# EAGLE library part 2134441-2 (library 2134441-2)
Body Features: Offset .88 MM | Shell Plating Material Tin over Nickel | Shell Plating Finish Matte | Connector Profile Micro | Configuration Features: Number of Positions 5 | Number of Ports 1 | Contact Features: Contact Mating Area Plating Material Thickness .76 MICM | Contact Current Rating (Max) 1.8 AMP | Contact Mating Area Plating Material Gold | Contact Mating Area Plating Material Thickness 29.52 MICIN | Dimensions: PCB Thickness (Recommended) .8 1. MM | PCB Thickness (Recommended) .031 .039 Source: Datasheet
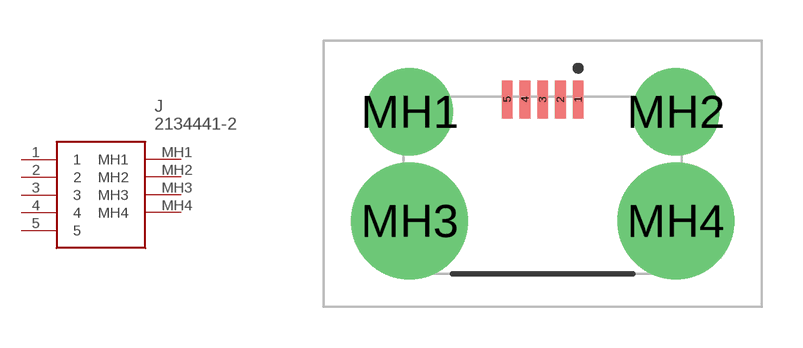
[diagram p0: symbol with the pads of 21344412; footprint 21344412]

Designator prefix J

## 2134441-2 (Arrow_Part_Number: 2134441-2; Arrow_Price-Stock: https://www.arrow.com/en/products/2134441-2/te-connectivity?region=nac; Description: Body Features: Offset .88 MM | Shell Plating Material Tin over Nickel | Shell Plating Finish Matte | Connector Profile Micro | Configuration Features: Number of Positions 5 | Number of Ports 1 | Contact Features: Contact Mating Area Plating Material Thickness .76 MICM | Contact Current Rating (Max) 1.8 AMP | Contact Mating Area Plating Material Gold | Contact Mating Area Plating Material Thickness 29.52 MICIN | Dimensions: PCB Thickness (Recommended) .8 1. MM | PCB Thickness (Recommended) .031 .039; Height: 1.9mm; Manufacturer_Name: TE Connectivity; Manufacturer_Part_Number: 2134441-2; Mouser_Part_Number: 571-2134441-2; Mouser_Price-Stock: https://www.mouser.co.uk/ProductDetail/TE-Connectivity/2134441-2?qs=kAqyOuzYGe%252Bz%252BAPK%2FThl2g%3D%3D)  [21344412]
1  1
2  2
3  3
4  4
5  5
MH1  MH1
MH2  MH2
MH3  MH3
MH4  MH4

## Footprint 21344412 (pad centres in mm)
2134441-2-3
smd 0.4 x 1.4: 1 1.3,4.45; 2 0.65,4.45; 3 0,4.45; 4 -0.65,4.45; 5 -1.3,4.45
drill 2.13 pad 3.195: MH1 -4.875,4; MH2 4.875,4
drill 2.86 pad 4.29: MH3 -4.875,0; MH4 4.875,0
